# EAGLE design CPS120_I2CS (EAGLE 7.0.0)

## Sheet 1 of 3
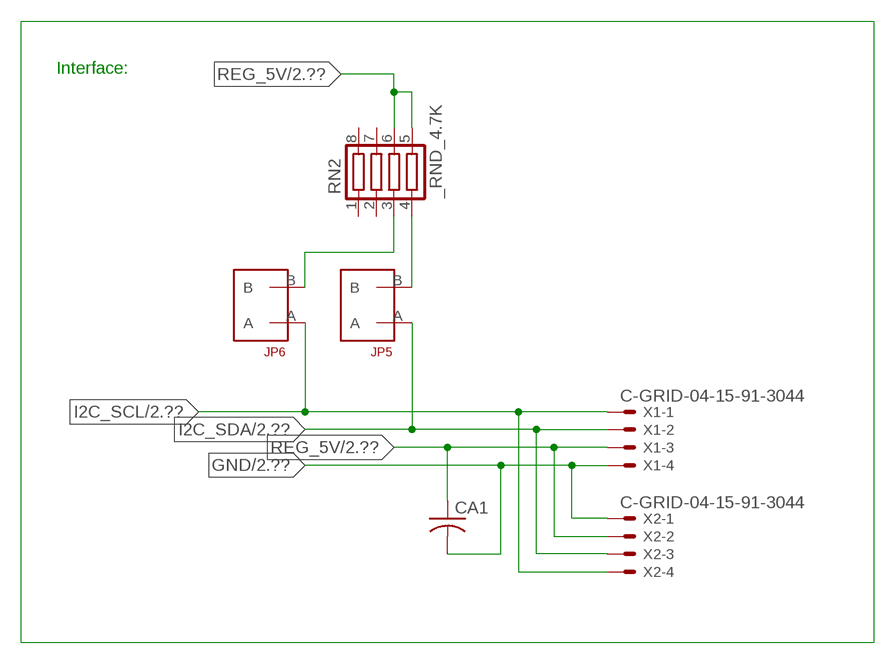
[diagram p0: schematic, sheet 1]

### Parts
CA1  CC1206KRX7R9BB104  [.1UF]
JP5  JUMPER_1X2_2MM  [JUMPER_1X2_2MM]
JP6  JUMPER_1X2_2MM  [JUMPER_1X2_2MM]
RN2  _RND_4.7K  [RND]
X1  C-GRID-04-15-91-3044  [15-91-04]
X2  C-GRID-04-15-91-3044  [15-91-04]

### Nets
GND: CA1.2 X1.4 X2.1 ; also sheet 2,3
I2C_SCL: JP6.A X1.1 X2.4 ; also sheet 2
I2C_SDA: JP5.A X1.2 X2.3 ; also sheet 2
N$1: JP6.B RN2.3
N$2: JP5.B RN2.4
REG_5V: CA1.1 RN2.5 RN2.6 X1.3 X2.2 ; also sheet 2,3
Unconnected: RN2.1 RN2.2 RN2.7 RN2.8

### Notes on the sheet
- Interface:

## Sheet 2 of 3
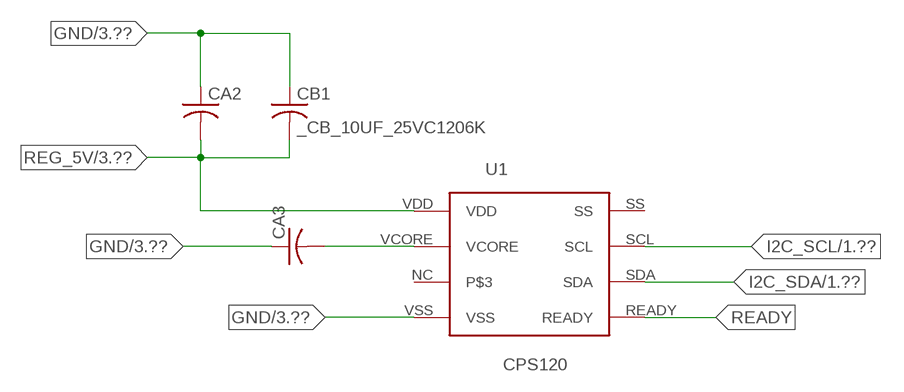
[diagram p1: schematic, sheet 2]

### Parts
CA2  _CA_.10UF_50VC1206K  [_CA_.1UF_50V]
CA3  _CA_.10UF_50VC1206K  [_CA_.1UF_50V]
CB1  _CB_10UF_25VC1206K  [_CB_10UF_25V]
U1  CPS120  [CPS120]

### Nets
GND: CA2.1 CA3.1 CB1.1 U1.VSS ; also sheet 1,3
I2C_SCL: U1.SCL ; also sheet 1
I2C_SDA: U1.SDA ; also sheet 1
N$6: CA3.2 U1.VCORE
READY: U1.READY
REG_5V: CA2.2 CB1.2 U1.VDD ; also sheet 1,3
Unconnected: U1.NC U1.SS

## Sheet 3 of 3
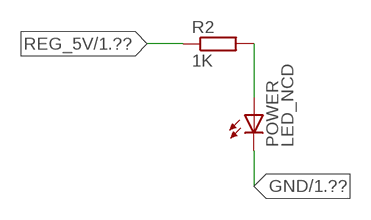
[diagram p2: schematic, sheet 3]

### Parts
POWER  LED_NCD  [CHIPLED_0603]
R2  1K  RESISTOR_SMT-0402  [R402]

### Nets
GND: POWER.C ; also sheet 1,2
N$3: POWER.A R2.2
REG_5V: R2.1 ; also sheet 1,2

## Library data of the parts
CA1 = NCD_ULTIMATE_LIBRARY:CC1206KRX7R9BB104: Capacitor CA .1uF 50V SMT C1206K CC1206KRX7R9BB104
CA2 CA3 = NCD_ULTIMATE_LIBRARY:_CA_.10UF_50V: Capacitor .1uF SMT
CB1 = NCD_ULTIMATE_LIBRARY:_CB_10UF_25V: Capacitor 10uF SMT
JP5 JP6 = NCD_ULTIMATE_CONNECTORS:JUMPER_1X2_2MM
POWER = NCD_ULTIMATE_LIBRARY:LED_NCD: LED Digikey 754-1132-2-ND/APT2012SRCPRV
R2 = NCD_ULTIMATE_LIBRARY:RESISTOR_SMT: NCD Resistor
RN2 = NCD_ULTIMATE_LIBRARY:_RND_4.7K: Resistor Array RND SMT 4.7K x 4 Single Resistor Source: http://www.ctscorp.com/components/Datasheets/CTSChipArrayDs.pdf Digikey 742C083472JPTR-ND/742C083472JP; OC_FARNELL: unknown; OC_NEWARK: unknown
U1 = NCD_ULTIMATE_bhaskar:CPS120
X1 X2 = NCD_ULTIMATE_CONNECTORS:C-GRID-04: CONNECTOR 4-Pos I2C wire to board 2.54 mm (0.100") pitch header Digikey WM1342-ND/0015912045; OC_FARNELL: unknown; OC_NEWARK: unknown

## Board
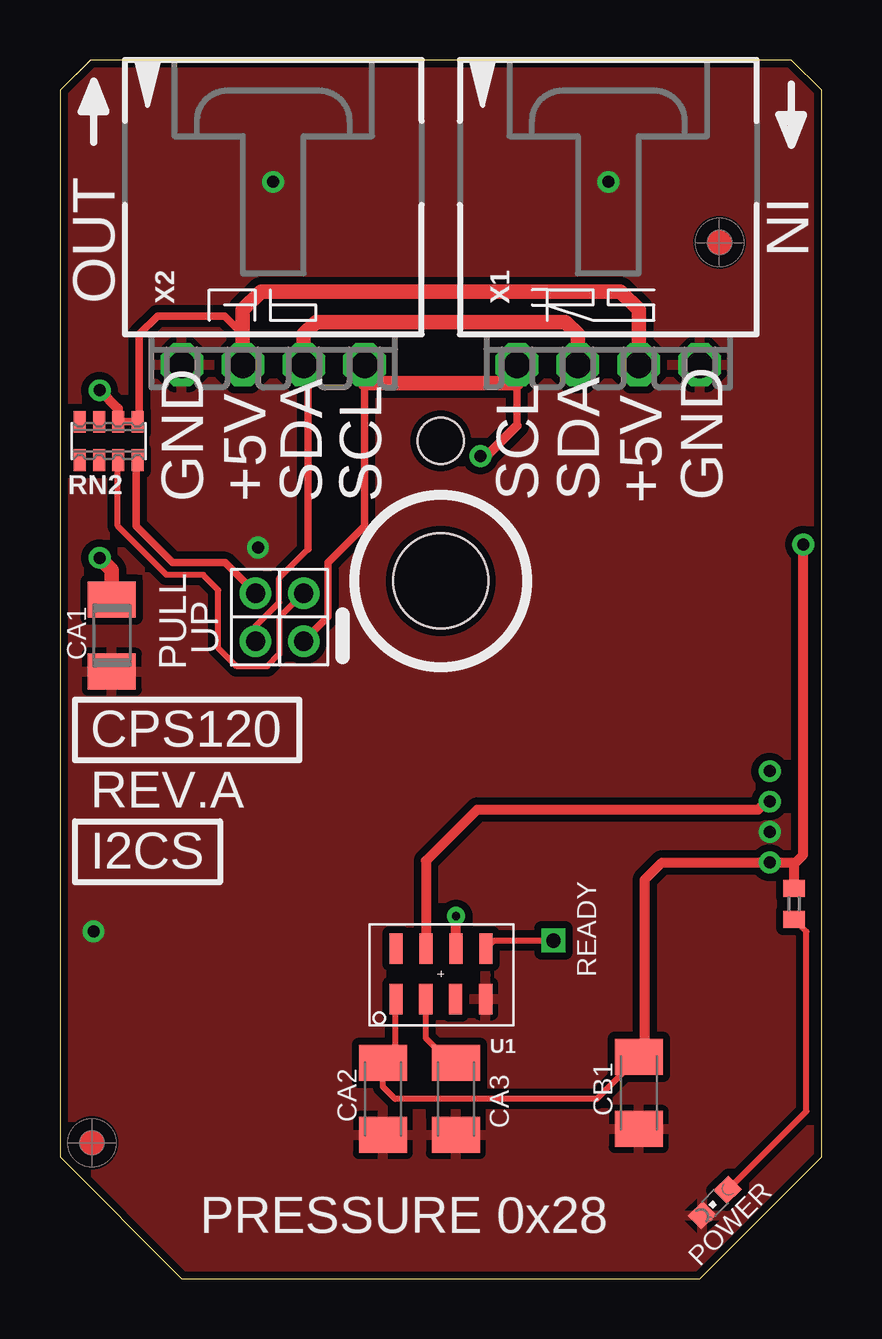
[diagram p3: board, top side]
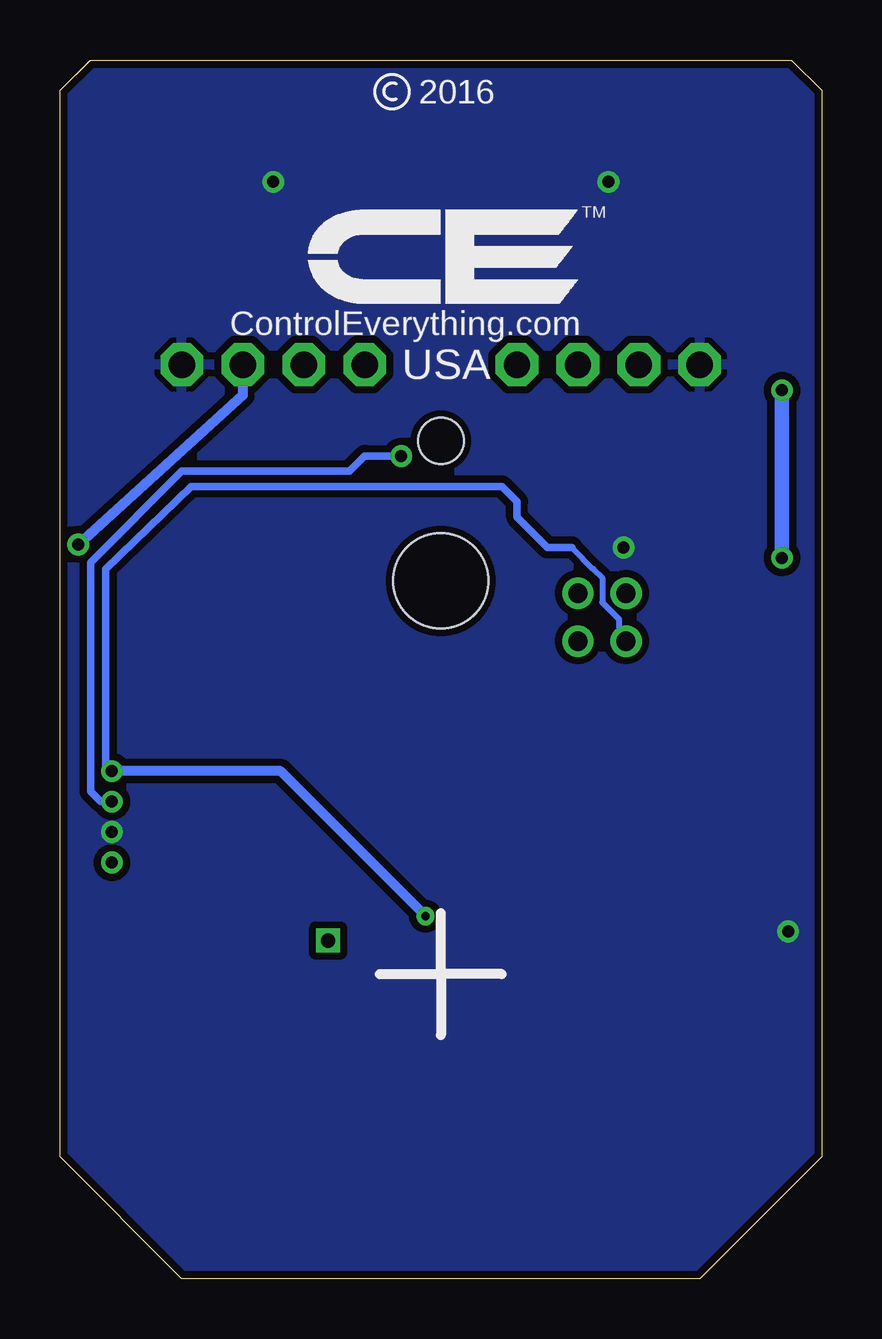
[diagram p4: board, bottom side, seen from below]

Size 31.75 x 50.8 mm. Coordinates in mm from the lower left corner, seen from the top.
Outline: 32 segments
Copper layers (1*16): Top 0.035mm / dielectric 1.5mm / Bottom 0.035mm
Design rules "default": minimum track width 5mil, minimum drill 24mil, track to track 5mil, track to pad 5mil, pad to pad 5mil, via to via 5mil, smd to smd 5mil, copper to edge 10mil, drill to drill 8mil, minimum pad ring 10mil, minimum via ring 8mil, stop-mask expansion 2mil, vias tented up to drill 0mil, thermal gap 10mil
Holes 3.96 mm at 15.88,29.08
Holes 1.91 mm at 15.88,34.92

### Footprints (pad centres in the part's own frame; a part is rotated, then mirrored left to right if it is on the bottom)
.1UF = smd 1.5 x 2: 1 -1.5,0; 2 1.5,0
_CA_.1UF_50V = smd 1.5 x 2: 1 -1.5,0; 2 1.5,0
_CB_10UF_25V = smd 1.5 x 2: 1 -1.5,0; 2 1.5,0
JUMPER_1X2_2MM = drill 0.8: A 0,2; B 0,0
CHIPLED_0603 = smd 0.8 x 0.876: A 0,-0.75; C 0,0.75
R402 = smd 0.7 x 0.9: 1 -0.65,0; 2 0.65,0
RND = smd 0.5 x 0.9: 1 -1.2,-0.8; 2 -0.4,-0.8; 3 0.4,-0.8; 4 1.2,-0.8; 5 1.2,0.8; 6 0.4,0.8; 7 -0.4,0.8; 8 -1.2,0.8
CPS120 = smd 0.55 x 1.27: NC 0.02,-2.9; READY -1.25,-5; SCL 1.25,-5; SDA 0,-5; SS 2.5,-5; VCORE 1.26,-2.9; VDD 2.5,-2.9; VSS -1.24,-2.9
15-91-04 = drill 1.1 pad 1.778 octagon: 1 -3.81,-7.62; 2 -1.27,-7.62; 3 1.27,-7.62; 4 3.81,-7.62

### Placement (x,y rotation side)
CA1  2.16,26.81 270 top
CA2  13.46,7.49 90 top
CA3  16.51,7.49 90 top
CB1  24.13,7.75 90 top
JP5  8.15,28.58 180 top
JP6  10.16,28.58 180 top
POWER  27.3,3.18 135 top
R2  30.61,15.62 270 top
RN2  2.03,34.92 0 top
U1  16.51,8.76 180 top
U$5  [VISION_REF10]  1.33,5.66 90 top
U$28  [VISION_REF10]  27.5,43.19 90 top
X1  22.86,45.72 0 top
X2  8.89,45.72 0 top

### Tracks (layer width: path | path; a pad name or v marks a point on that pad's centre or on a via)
GND  (via drill 0.5)
  other vias: 8.89,45.72 22.86,45.72 29.59,18.62 1.4,14.48 8.26,30.48
  pour Bottom (isolate 0.305): 4.45,-0.63 -0.63,4.45 -0.63,50.17 0.64,51.44 31.12,51.44 32.38,50.17 32.38,4.45 27.3,-0.63
  pour Top (isolate 0.305): 3.81,-1.27 -1.27,3.81 -1.27,50.8 0,52.07 31.75,52.07 33.02,50.8 33.02,3.81 27.94,-1.27
I2C_SCL  (via drill 0.5)
  Top 0.305: JP6.A 11.18,27.61 11.18,29.85 12.7,31.37 X2.4 | 19.05,35.56 X1.1
  Top 0.406: X2.4 12.7,37.34 | 19.05,37.34 X1.1 | v29.59,19.89 29.44,19.89 29.11,19.56 17.4,19.56 15.26,17.42 U1.SCL | 19.05,35.56 17.78,34.29 v17.53,34.29
  Top 0.61: 12.7,37.34 19.05,37.34
  Bottom 0.305: v29.59,19.89 30.05,19.89 30.48,20.32 30.48,29.85 26.67,33.66 19.69,33.66 19.05,34.29 v17.53,34.29
I2C_SDA  (via drill 0.35, 0.5)
  Top 0.254: JP5.A 8.15,27.2 9.14,28.19 9.14,29.21 10.35,30.42
  Top 0.305: 10.35,30.42 10.35,37.91 X2.3
  Top 0.406: U1.SDA v16.51,15.11
  Top 0.61: X2.3 10.16,39.37 10.67,39.88 21.08,39.88 21.59,39.37 X1.2
  Bottom 0.254: 10.41,30.48 9.52,29.59 9.14,29.21 9.14,28.19 8.45,27.5 8.45,26.87 JP5.A
  Bottom 0.305: 10.41,30.48 11.43,30.48 12.7,31.75 12.7,32.39 13.34,33.02 26.29,33.02 29.85,29.59 29.85,21.41 v29.59,21.16
  Bottom 0.406: v16.51,15.11 22.55,21.16 v29.59,21.16
N$1
  Top 0.254: JP6.B | JP6.B 9.14,27.56 9.14,26.04 8.64,25.53 7.37,25.53 6.6,26.29 6.6,28.7 5.97,29.34 4.45,29.34 2.41,31.37 2.41,34.11 RN2.3
N$2
  Top 0.305: JP5.B 6.88,29.85 4.7,29.85 3.18,31.37 3.18,34.07 RN2.4
N$3
  Top 0.254: POWER.A 31.12,6.99 31.12,14.46 R2.2
N$6
  Top 0.254: U1.VCORE 15.24,11.65 15.24,10.03 16.28,8.99 CA3.2
READY  (via drill 0.6)
  Top 0.254: U1.READY 18.09,14.1 v20.57,14.1
REG_5V  (via drill 0.5)
  Top 0.254: U1.VDD 13.97,11.62 13.97,9.01 | CB1.2 22.38,7.49 13.97,7.49 13.46,8 CA2.2
  Top 0.305: 7.62,39.37 7.49,39.37 | RN2.6 RN2.5 3.3,35.8 3.3,39.37 4.06,40.13 6.86,40.13 7.62,39.37 | X2.2 7.62,39.37
  Top 0.406: 30.48,17.35 v29.59,17.35 25.1,17.35 24.38,16.64 24.38,9.5 CB1.2 | 30.48,17.35 30.67,17.35 30.99,17.67 v30.99,30.61 | v1.65,37.03 2.41,36.27 2.41,35.74 RN2.6 | 13.46,9.02 14.22,9.02 13.97,9.01 CA2.2 | R2.1 30.61,17.22 30.48,17.35
  Top 0.61: X1.3 24.13,40.39 23.37,41.15 8.38,41.15 7.62,40.39 X2.2 | CA1.1 2.16,29.54 v1.65,30.05
  Bottom 0.406: v30.99,30.61 24.13,36.83 24.13,37.47 24.16,38.08 24.13,38.23 X1.3
  Bottom 0.61: v1.65,30.05 v1.65,37.03

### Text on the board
tNames: IN | OUT | GND | +5V | SDA | SCL | SCL | SDA | +5V | GND | UP | PULL | CPS120 | REV.A | I2CS | READY | PRESSURE 0x28
bNames: 2016 | TM | ControlEverything.com | USA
